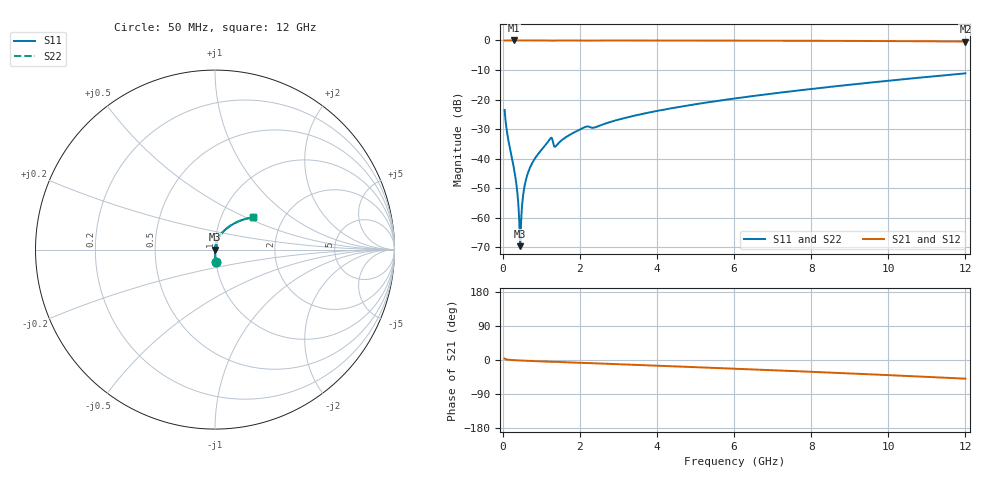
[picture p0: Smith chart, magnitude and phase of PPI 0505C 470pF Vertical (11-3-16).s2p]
# GHz S MA R 50
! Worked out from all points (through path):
!   1601 points, 50 MHz to 12 GHz, reference 50 ohm
!   highest |S21| = 0.00 dB at 296.5 MHz (marker M1); lowest = -0.4 dB at 12 GHz (marker M2)
!   group delay of S21, straight-line fit = 11.4 ps
!   lowest |S11| = -69.6 dB at 453.3 MHz (marker M3), VSWR 1.00, Z = 50 - j0.000883 ohm
!   |S11| at or under -10 dB: start of sweep to end of sweep
!   |S22| runs from -69.6 to -11.1 dB; largest |S21 - S12| = 0
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0.05  0.06669 -86.2  0.9976 3.7  0.9976 3.7  0.06669 -86.2
0.1545625  0.01935 -88.6  0.9996 0.7  0.9996 0.7  0.01935 -88.6
0.2964688  0.006554 -88.0  0.9997 -0.5  0.9997 -0.5  0.006554 -88.0
0.3562187  0.00366 -86.0  0.9997 -0.8  0.9997 -0.8  0.00366 -86.0
0.4159687  0.001332 -77.2  0.9997 -1.1  0.9997 -1.1  0.001332 -77.2
0.4533125  0.0003295 -1.5  0.9996 -1.3  0.9996 -1.3  0.0003295 -1.5
0.4906563  0.001238 72.6  0.9996 -1.5  0.9996 -1.5  0.001238 72.6
0.5504062  0.002965 81.4  0.9996 -1.7  0.9996 -1.7  0.002965 81.4
0.617625  0.004769 83.5  0.9996 -2.0  0.9996 -2.0  0.004769 83.5
0.7221875  0.007366 84.4  0.9995 -2.5  0.9995 -2.5  0.007366 84.4
0.8640937  0.01069 84.5  0.9994 -3.1  0.9994 -3.1  0.01069 84.5
1.222594  0.02138 76.2  0.9963 -4.7  0.9963 -4.7  0.02138 76.2
1.386906  0.01644 74.4  0.9967 -4.9  0.9967 -4.9  0.01644 74.4
1.625906  0.02276 81.5  0.9986 -5.9  0.9986 -5.9  0.02276 81.5
2.044156  0.03212 79.2  0.9976 -7.7  0.9976 -7.7  0.03212 79.2
2.387719  0.03369 75.4  0.9958 -8.7  0.9958 -8.7  0.03369 75.4
3.067375  0.04688 77.4  0.9977 -11.4  0.9977 -11.4  0.04688 77.4
4.038312  0.06474 74.0  0.9967 -15.2  0.9967 -15.2  0.06474 74.0
6.025  0.1043 66.4  0.9932 -23.0  0.9932 -23.0  0.1043 66.4
8.019156  0.1513 58.3  0.9868 -31.2  0.9868 -31.2  0.1513 58.3
10.01331  0.2083 49.7  0.9761 -39.9  0.9761 -39.9  0.2083 49.7
12  0.2773 40.4  0.9584 -49.3  0.9584 -49.3  0.2773 40.4
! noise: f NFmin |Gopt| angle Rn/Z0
0.05  0.0002979  0.8265  0.2125  0.000361
1.372  0.007088  0.8026  3.89  0.007444
2.701  0.006108  0.6003  7.383  0.002805
4.031  0.0064  0.4765  10.37  0.002063
5.36  0.007704  0.4388  13.3  0.002248
6.682  0.009068  0.4178  16.04  0.002501
8.012  0.01049  0.4059  18.66  0.002796
9.341  0.01198  0.401  21.15  0.003137
10.67  0.01357  0.402  23.56  0.003538
12  0.0153  0.4082  25.94  0.004017
